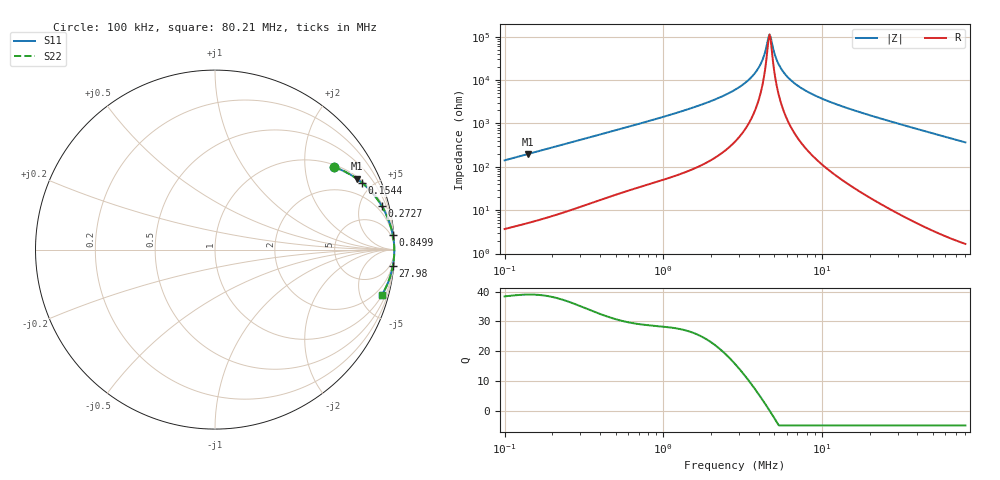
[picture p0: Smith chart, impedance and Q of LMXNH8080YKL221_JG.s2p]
! LMXNH8080YKL221_JG  S-PARAMETER MODEL  ( Standard Model )
! Model Generated by TAIYO YUDEN Corporation (https://www.yuden.co.jp/en/)
! Version 1.0
! TAIYO YUDEN Control No. 20250523
! Copyright(c) 2025 TAIYO YUDEN CO.,LTD. All Rights Reserved.
! Product Description (link to TY-COMPAS)
! https://ds.yuden.co.jp/TYCOMPAS/or/detail?pn=LMXNH8080YKL221MJG&u=M
! Products Name : Inductors
! Characteristics :
!  Inductance : 220 [uH] , SRF(min) : 4.0 [MHz] , DC Resistance(max) : 0.806 [Ohm]
!  Rated Current : Saturation  700 [mA] , Temp Rise  670 [mA] (40 [degC])
!  Case Size : 8.0 x 8.0 / 0.315 x 0.315 [mm/inch] , Thickness : 4.0 / 0.157 [mm/inch]
!  (Conditions: Temperature = 25 [degC] , DC Bias Current = 0 [A])
! External Node Assignments :
!  1  o---GGG---o  2
! GND o---------o GND
! Frequency Range : 0.1MHz  -  80.209071MHz  [ 402 STEP ]
# MHz S RI R 50
! Freq[MHz].  S11 Real  S11 Imag  S21 Real  S21 Imag  S12 Real  S12 Imag  S22 Real  S22 Imag
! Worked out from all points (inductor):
!   401 points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, 100 kHz to 80.21 MHz, reference 50 ohm
!   read as one part in series: L = 224 uH near 103.4 kHz
!   highest Q = 39.1 at 139.7 kHz (marker M1), where L = 224 uH
!   self-resonance near 4.677 MHz
!   S11 on the Smith chart (normalised r, x): 100 kHz: 1.07, +2.83; 154.4 kHz: 1.11, +4.34; 272.7 kHz: 1.21, +7.63; 849.9 kHz: 2, +24; 27.98 MHz: 1, -22; 80.21 MHz: 1.03, -7.34
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0.1  0.6625 0.46  0.3375 -0.46  0.3375 -0.46  0.6625 0.46
0.139705  0.7886 0.3957  0.2114 -0.3957  0.2114 -0.3957  0.7886 0.3957
0.154445  0.8188 0.3726  0.1812 -0.3726  0.1812 -0.3726  0.8188 0.3726
0.272668  0.9298 0.2419  0.0702 -0.2419  0.0702 -0.2419  0.9298 0.2419
0.306519  0.9427 0.2185  0.0573 -0.2185  0.0573 -0.2185  0.9427 0.2185
0.849868  0.9902 0.0824  0.00977 -0.0824  0.00977 -0.0824  0.9902 0.0824
0.939539  0.9918 0.0743  0.0082 -0.0743  0.0082 -0.0743  0.9918 0.0743
1.864652  0.9975 0.0334  0.00251 -0.0334  0.00251 -0.0334  0.9975 0.0334
2.832121  0.9987 0.0166  0.00133 -0.0166  0.00133 -0.0166  0.9987 0.0166
3.403909  0.9989 0.0103  0.00108 -0.0103  0.00108 -0.0103  0.9989 0.0103
3.89101  0.999 0.00589  0.000964 -0.00589  0.000964 -0.00589  0.999 0.00589
4.230241  0.9991 0.00321  0.000916 -0.00321  0.000916 -0.00321  0.9991 0.00321
4.5228  0.9991 0.00107  0.000891 -0.00107  0.000891 -0.00107  0.9991 0.00107
4.676581  0.9991 9.67e-06  0.000883 -9.67e-06  0.000883 -9.67e-06  0.9991 9.67e-06
4.835592  0.9991 -0.00105  0.000878 0.00105  0.000878 0.00105  0.9991 -0.00105
5.257175  0.9991 -0.00372  0.000875 0.00372  0.000875 0.00372  0.9991 -0.00372
5.811868  0.9991 -0.00696  0.000895 0.00696  0.000895 0.00696  0.9991 -0.00696
6.86944  0.999 -0.0125  0.000985 0.0125  0.000985 0.0125  0.999 -0.0125
8.680988  0.9987 -0.021  0.00125 0.021  0.00125 0.021  0.9987 -0.021
26.60888  0.9915 -0.0871  0.00848 0.0871  0.00848 0.0871  0.9915 -0.0871
27.97746  0.9907 -0.0918  0.00934 0.0918  0.00934 0.0918  0.9907 -0.0918
80.20907  0.9298 -0.2531  0.0702 0.2531  0.0702 0.2531  0.9298 -0.2531
